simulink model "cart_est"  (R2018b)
settings: Solver=ode4  StartTime=0.0  StopTime=10.0  FixedStep=1e-3  RelTol=1e-3
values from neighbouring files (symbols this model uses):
  k_1 = 1 / m    (= 0.695894224078)    [mainSkript_modifikaceVozik.m]    (also in mainSkript_estimaceVozik.m = 1 / m; mainSkript_odhadKyvadlaZvlast.m = params.k_1; mainSkript_kyvadlaNajednouOdhad.m = params.k_1)
  kn = bn_0 / m    [mainSkript_modifikaceVozik.m]    (also in mainSkript_estimaceVozik.m)
  kns = bs_n / m    (= 4.77362560891)    [mainSkript_modifikaceVozik.m]
  kp = bp_0 / m    (= 1.28051496173)    [mainSkript_modifikaceVozik.m]    (also in mainSkript_estimaceVozik.m = bp_0 / m)
  kps = bs_p / m    (= 3.81746694502)    [mainSkript_modifikaceVozik.m]
  v_0 = v(1)    [mainSkript_modifikaceVozik.m]    (also in mainSkript_estimaceVozik.m = v(n_start))
  x_0 = x(1)    [mainSkript_modifikaceVozik.m]    (also in mainSkript_estimaceVozik.m = x(n_start))
libraries: simulink x2

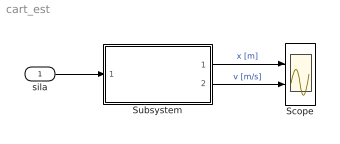
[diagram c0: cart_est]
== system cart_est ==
  sila : Inport
  Scope : Scope  NumInputPorts=2
  Subsystem : Subsystem
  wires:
  Subsystem/1(x) -> Scope/1  "x [m]"
  sila/1 -> Subsystem/1(sila [N])
  Subsystem/2(v) -> Scope/2  "v [m/s]"

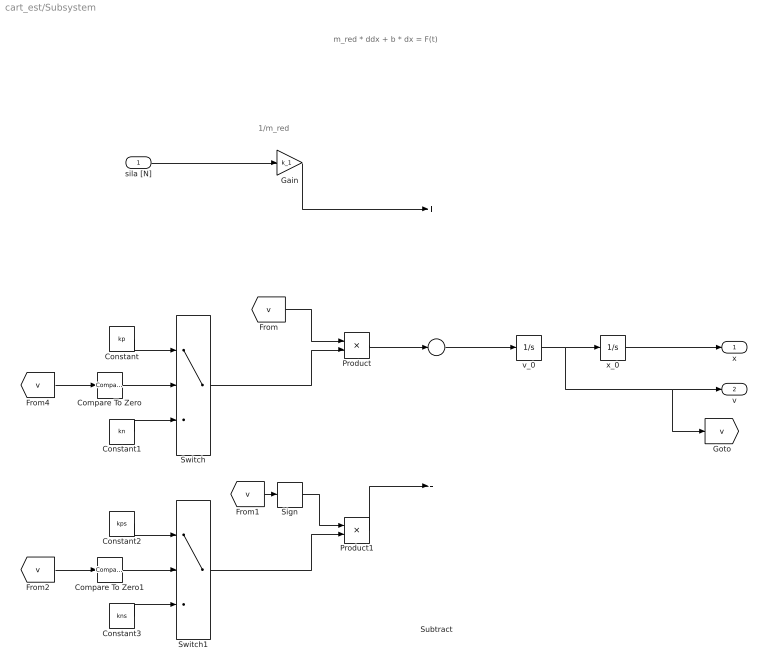
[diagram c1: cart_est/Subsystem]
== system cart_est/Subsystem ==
  note: 1/m_red
  note: m_red * ddx + b * dx = F(t)
  sila [N] : Inport
  Compare To Zero : simulink/Logic and Bit Operations/Compare To Zero  relop=>  OutDataTypeStr=boolean
  Compare To Zero1 : simulink/Logic and Bit Operations/Compare To Zero  relop=>  OutDataTypeStr=boolean
  Constant : Constant  Value=kp
  Constant1 : Constant  Value=kn
  Constant2 : Constant  Value=kps
  Constant3 : Constant  Value=kns
  Gain : Gain  Gain=k_1
  Product : Product
  Product1 : Product
  Sign : Signum
  Subtract : Sum  Inputs=+--
  Switch : Switch  Criteria=u2 > Threshold
  Switch1 : Switch  Criteria=u2 > Threshold
  v_0 : Integrator  InitialCondition=v_0
  x_0 : Integrator  InitialCondition=x_0
  x : Outport
  v : Outport  Port=2
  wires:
  Product/1 -> Subtract/2
  x_0/1 -> x/1
  [v] -> Product/1
  Constant1/1 -> Switch/3
  Compare To Zero/1 -> Switch/2
  [v] -> Compare To Zero/1
  Constant/1 -> Switch/1
  Switch/1 -> Product/2
  v_0/1 -> v/1, [v], x_0/1
  sila [N]/1 -> Gain/1
  Subtract/1 -> v_0/1
  Gain/1 -> Subtract/1
  Switch1/1 -> Product1/2
  Constant2/1 -> Switch1/1
  [v] -> Compare To Zero1/1
  Compare To Zero1/1 -> Switch1/2
  Constant3/1 -> Switch1/3
  Product1/1 -> Subtract/3
  [v] -> Sign/1
  Sign/1 -> Product1/1
